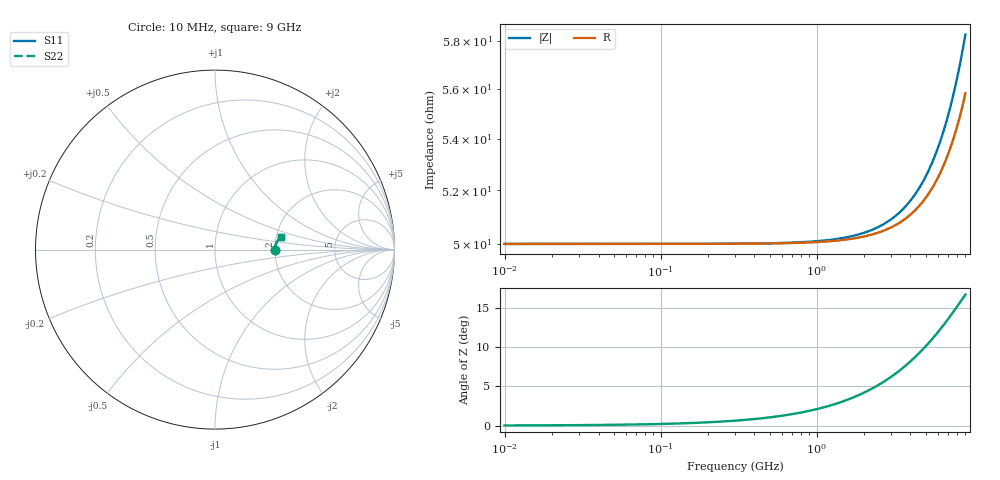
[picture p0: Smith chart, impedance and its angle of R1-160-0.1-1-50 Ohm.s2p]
!version-2
!date-03.2021
# MHz S RI R 50
!Freq ReS11 ImS11 ReS21 ImS21 ReS12 ImS12 ReS22 ImS22
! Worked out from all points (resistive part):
!   451 points, 10 MHz to 9 GHz, reference 50 ohm
!   read as one part in series: R = 50 ohm at 50 MHz
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10  0.3333 8.13e-05  0.6667 -8.13e-05  0.6667 -8.13e-05  0.3333 8.13e-05
50  0.3333 0.000407  0.6667 -0.000407  0.6667 -0.000407  0.3333 0.000407
390  0.3334 0.00317  0.6666 -0.00317  0.6666 -0.00317  0.3334 0.00317
750  0.3336 0.0061  0.6664 -0.0061  0.6664 -0.0061  0.3336 0.0061
1130  0.3338 0.00918  0.6662 -0.00918  0.6662 -0.00918  0.3338 0.00918
1510  0.3342 0.0123  0.6658 -0.0123  0.6658 -0.0123  0.3342 0.0123
1870  0.3347 0.0152  0.6653 -0.0152  0.6653 -0.0152  0.3347 0.0152
2250  0.3353 0.0182  0.6647 -0.0182  0.6647 -0.0182  0.3353 0.0182
2630  0.3361 0.0213  0.6639 -0.0213  0.6639 -0.0213  0.3361 0.0213
3010  0.3369 0.0243  0.6631 -0.0243  0.6631 -0.0243  0.3369 0.0243
3370  0.3378 0.0271  0.6622 -0.0272  0.6622 -0.0272  0.3378 0.0271
3750  0.3389 0.0301  0.6611 -0.0302  0.6611 -0.0302  0.3389 0.0301
4130  0.3401 0.0331  0.6599 -0.0331  0.6599 -0.0331  0.3401 0.0331
4510  0.3414 0.0361  0.6586 -0.0361  0.6586 -0.0361  0.3414 0.0361
4870  0.3427 0.0388  0.6573 -0.0388  0.6573 -0.0388  0.3427 0.0388
5250  0.3443 0.0417  0.6557 -0.0417  0.6557 -0.0417  0.3443 0.0417
5630  0.3459 0.0446  0.6541 -0.0446  0.6541 -0.0446  0.3459 0.0446
6010  0.3477 0.0474  0.6523 -0.0474  0.6523 -0.0474  0.3477 0.0474
6750  0.3514 0.0528  0.6486 -0.0528  0.6486 -0.0528  0.3514 0.0528
7510  0.3557 0.0582  0.6443 -0.0582  0.6443 -0.0582  0.3557 0.0582
8210  0.3601 0.063  0.6399 -0.063  0.6399 -0.063  0.3601 0.063
9000  0.3655 0.0681  0.6345 -0.0682  0.6345 -0.0682  0.3655 0.0681
